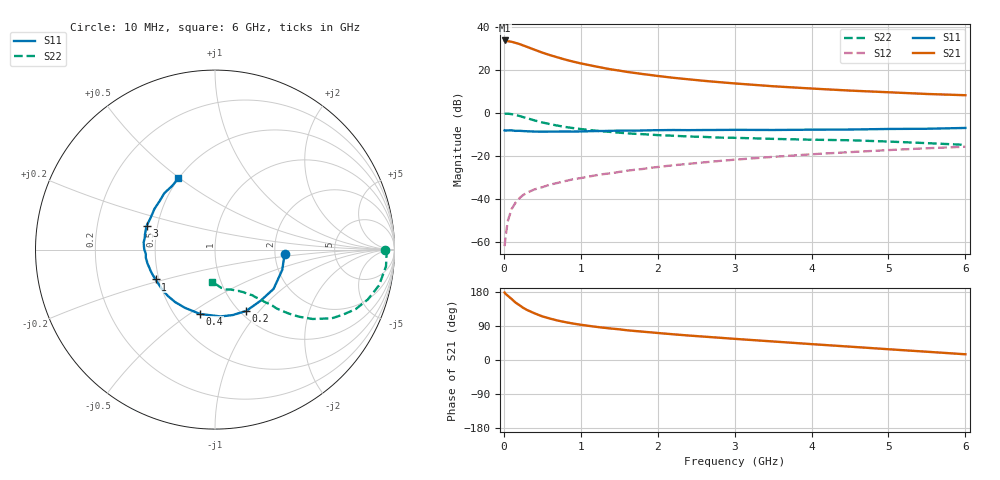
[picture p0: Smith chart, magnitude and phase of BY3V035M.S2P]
! SIEMENS Small Signal Semiconductors
! BFY420
! Si NPN RF SIEGET Grounded Emitter Transistor in MICRO-X
! VCE = 3 V  IC = 35 mA
! Common Emitter S-Parameters:  October  1996
# GHz  S  MA  R  50
!  f  S11  S21  S12  S22
! GHz  MAG  ANG  MAG  ANG  MAG  ANG  MAG  ANG
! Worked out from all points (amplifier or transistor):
!   36 points, 10 MHz to 6 GHz, reference 50 ohm
!   highest |S21| = 33.6 dB at 10 MHz (marker M1)
!   |S21| within 3 dB of that: start of sweep to 302.8 MHz
!   unconditionally stable (mu >= 1): start of sweep to 10.99 MHz; 1.588 GHz to end of sweep
!   at 250 MHz: K = 0.38, MSG = 34.8 dB, |S12| = -38.2 dB
!   at 1.4 GHz: K = 0.98, MSG = 24.1 dB, |S12| = -28.0 dB
!   at 6 GHz: K = 1.06, MAG = 10.5 dB, |S12| = -15.7 dB
!   S11 on the Smith chart (normalised r, x): 10 MHz: 2.28, -0.13; 200 MHz: 1.07, -0.86; 400 MHz: 0.66, -0.55; 1 GHz: 0.48, -0.18; 3 GHz: 0.43, +0.14; 6 GHz: 0.50, +0.49
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0.01  0.3926 -3.5  48.11 178.1  0.0008 110.9  0.9449 0.0
0.02  0.3875 -6.5  47.53 175.0  0.0012 89.1  0.9562 -1.4
0.1  0.393 -33.8  44.88 161.2  0.0058 80.7  0.9353 -12.3
0.15  0.3818 -48.4  42.35 151.9  0.0081 72.9  0.8955 -18.1
0.2  0.3834 -63.0  39.86 145.0  0.0103 71.2  0.8504 -23.0
0.25  0.3778 -74.9  36.93 137.9  0.0123 68.2  0.798 -27.1
0.3  0.3737 -85.3  34.21 132.1  0.014 67.4  0.7546 -30.5
0.4  0.3681 -103.0  29.29 123.1  0.0167 65.0  0.6673 -35.4
0.5  0.3651 -117.3  25.09 115.1  0.0188 64.2  0.5994 -38.6
0.6  0.3672 -127.1  21.96 109.3  0.0215 63.5  0.5467 -40.8
0.7  0.3682 -135.3  19.43 104.1  0.0236 62.9  0.5051 -42.5
0.8  0.3694 -142.9  17.25 99.9  0.0261 62.0  0.4705 -43.8
1  0.3703 -153.3  14.1 93.0  0.0306 64.0  0.4213 -45.4
1.1  0.3741 -157.4  12.97 90.2  0.033 64.2  0.4018 -46.5
1.4  0.384 -168.1  10.2 82.9  0.0396 64.8  0.3594 -48.7
1.6  0.3883 -173.5  8.965 78.5  0.0453 63.8  0.3355 -50.3
2.2  0.3996 174.1  6.54 67.9  0.0606 61.4  0.2947 -55.1
3  0.4035 161.0  4.832 55.8  0.0817 56.7  0.2634 -61.3
3.5  0.4001 153.2  4.152 48.9  0.0951 53.3  0.2487 -65.2
4.5  0.4101 138.9  3.293 35.2  0.1225 44.9  0.2311 -73.9
5.5  0.4276 124.0  2.748 21.8  0.1507 35.6  0.198 -86.6
6  0.4463 117.2  2.57 15.1  0.1636 30.7  0.1805 -95.2
